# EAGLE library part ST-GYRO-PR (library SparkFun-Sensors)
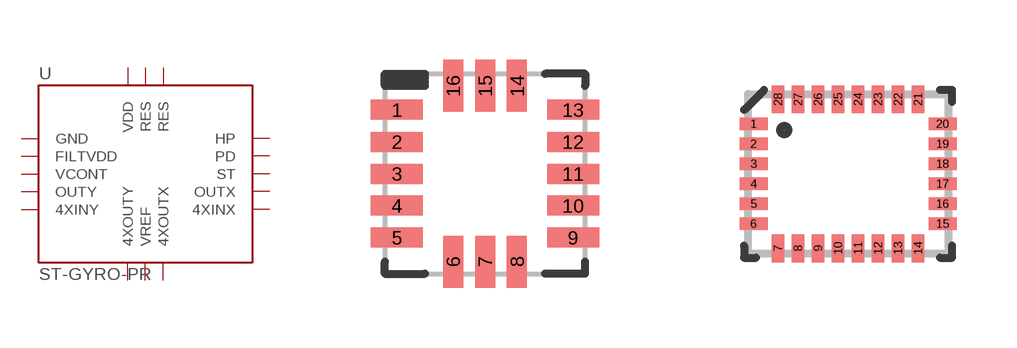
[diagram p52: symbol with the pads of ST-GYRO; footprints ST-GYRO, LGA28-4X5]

Designator prefix -

## ST-GYRO-PRLGA  [ST-GYRO]
1  GND
2  FILTVDD
3  VCONT
4  OUTY
5  4XINY
6  4XOUTY
7  VREF
8  4XOUTX
9  4XINX
10  OUTX
11  ST
12  PD
13  HP
14  RES
15  RES
16  VDD

## ST-GYRO-PRLGA28  [LGA28-4X5]
1  OUTX
5  4XINX
7  4XOUTX
9  VDD
14  4XOUTY
16  4XINY
17  VCONT
18  FILTVDD
19  RES
20  OUTY
22  VREF
24  HP
25  RES
26  GND
27  ST
28  PD

## Footprint ST-GYRO (pad centres in mm)
smd 1.3 x 0.5: 1 -2.2,1.6; 2 -2.2,0.8; 3 -2.2,0; 4 -2.2,-0.8; 5 -2.2,-1.6; 9 2.2,-1.6; 10 2.2,-0.8; 11 2.2,0; 12 2.2,0.8; 13 2.2,1.6
smd 0.5 x 1.3: 6 -0.8,-2.2; 7 0,-2.2; 8 0.8,-2.2; 14 0.8,2.2; 15 0,2.2; 16 -0.8,2.2

## Footprint LGA28-4X5 (pad centres in mm)
smd 0.7 x 0.31: 1 -2.362,1.25; 2 -2.362,0.75; 3 -2.362,0.25; 4 -2.362,-0.25; 5 -2.362,-0.75; 6 -2.362,-1.25; 15 2.362,-1.25; 16 2.362,-0.75; 17 2.362,-0.25; 18 2.362,0.25; 19 2.362,0.75; 20 2.362,1.25
smd 0.31 x 0.7: 7 -1.75,-1.863; 8 -1.25,-1.863; 9 -0.75,-1.863; 10 -0.25,-1.863; 11 0.25,-1.863; 12 0.75,-1.863; 13 1.25,-1.863; 14 1.75,-1.863; 21 1.75,1.863; 22 1.25,1.863; 23 0.75,1.863; 24 0.25,1.863; 25 -0.25,1.863; 26 -0.75,1.863; 27 -1.25,1.863; 28 -1.75,1.863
